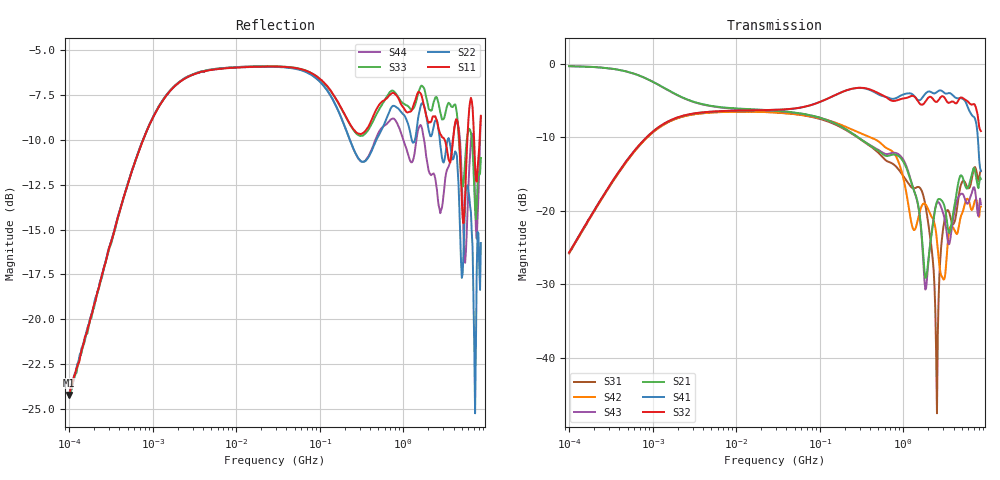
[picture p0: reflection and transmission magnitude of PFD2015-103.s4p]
# MHz S MA R 50
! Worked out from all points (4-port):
!   498 points, 100 kHz to 8.5 GHz, reference 50 ohm
!   strongest paths, dB at 100 kHz, 1.698 MHz, 29.49 MHz, 500.7 MHz, 8.5 GHz:
!     S32: -25.7, -7.6, -6.3, -4.0, -9.2
!     S41: -25.7, -7.6, -6.3, -4.2, -14.6
!     S21: -0.3, -3.9, -6.4, -11.8, -15.7
!     S43: -0.3, -3.9, -6.4, -11.7, -19.1
!     S42: -25.8, -7.7, -6.6, -10.5, -19.4
!     S31: -25.8, -7.7, -6.6, -12.1, -14.6
!   lowest |S11| = -24.2 dB at 100 kHz (marker M1), VSWR 1.13, Z = 53.3 + j5.44 ohm
!   |S11| at or under -10 dB: 3.129 GHz to 3.948 GHz (818.8 MHz wide, 23.1 % of centre); 4.694 GHz to 5.852 GHz (1.159 GHz wide, 22 % of centre); 7.056 GHz to 8.201 GHz (1.146 GHz wide, 15 % of centre)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
0.1  0.06144 55.8  0.9609 -3.1  0.05153 -97.3  0.05197 82.9
     0.9609 -3.1  0.06182 55.4  0.05218 82.1  0.05145 -97.5
     0.05153 -97.3  0.05218 82.1  0.06061 54.0  0.9605 -3.1
     0.05197 82.9  0.05145 -97.5  0.9605 -3.1  0.0615 55.0
90.29583  0.4771 -22.1  0.4369 -49.3  0.4278 133.0  0.5366 -0.5
          0.4369 -49.3  0.4701 -25.1  0.5365 -0.7  0.4321 129.5
          0.4278 133.0  0.5365 -0.7  0.4768 -21.9  0.4361 -49.1
          0.5366 -0.5  0.4321 129.5  0.4361 -49.1  0.4709 -25.2
1306.515  0.391 -177.6  0.1437 -136.2  0.1427 15.5  0.6153 -171.7
          0.1437 -136.2  0.3105 -178.0  0.6031 -171.4  0.07582 23.4
          0.1427 15.5  0.6031 -171.4  0.3858 -176.1  0.1446 -140.5
          0.6153 -171.7  0.07582 23.4  0.1446 -140.5  0.2772 178.2
2533.649  0.3575 28.6  0.1156 135.8  0.004216 156.8  0.6419 32.2
          0.1156 135.8  0.3589 27.5  0.5504 34.2  0.06259 33.7
          0.004216 156.8  0.5504 34.2  0.4149 29.8  0.1135 119.6
          0.6419 32.2  0.06259 33.7  0.1135 119.6  0.2292 14.2
4000.492  0.3267 -133.7  0.09927 -63.7  0.08156 -59.9  0.6032 -167.5
          0.09927 -63.7  0.2806 -147.7  0.5507 -157.6  0.07629 -120.6
          0.08156 -59.9  0.5507 -157.6  0.3942 -155.1  0.09135 -71.9
          0.6032 -167.5  0.07629 -120.6  0.09135 -71.9  0.3282 -136.7
5383.342  0.1959 1.9  0.1546 85.7  0.1587 100.8  0.5656 6.3
          0.1546 85.7  0.1822 -25.8  0.574 19.7  0.1079 61.8
          0.1587 100.8  0.574 19.7  0.2553 -7.5  0.1236 80.7
          0.5656 6.3  0.1079 61.8  0.1236 80.7  0.1485 40.2
8500  0.3693 -31.3  0.1647 32.8  0.1864 44.3  0.1867 -46.1
      0.1647 32.8  0.163 -27.8  0.3484 -38.5  0.1068 -4.2
      0.1864 44.3  0.3484 -38.5  0.2816 -42.7  0.1111 33.9
      0.1867 -46.1  0.1068 -4.2  0.1111 33.9  0.368 -21.8
